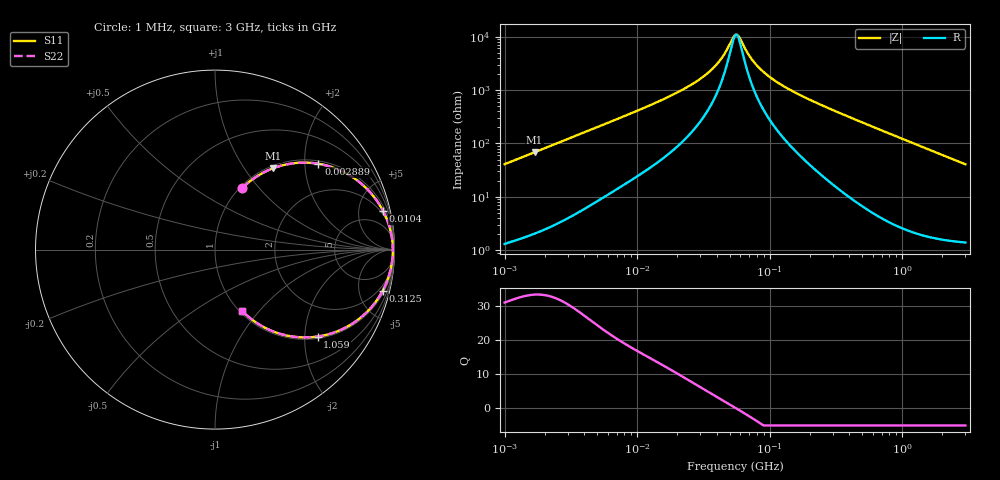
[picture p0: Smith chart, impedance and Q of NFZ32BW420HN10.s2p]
! NFZ32BW420HN10
# Hz S RI R 50
!Freq.(Hz) S11(Real) S11(Imag) S21(Real) S21(Imag) S12(Real) S12(Imag) S22(Real) S22(Imag)
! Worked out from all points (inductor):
!   401 points, 1 MHz to 3 GHz, reference 50 ohm
!   read as one part in series: L = 6.49 uH near 1.041 MHz
!   highest Q = 33.4 at 1.683 MHz (marker M1), where L = 6.48 uH
!   self-resonance near 55.88 MHz
!   S11 on the Smith chart (normalised r, x): 1 MHz: 1.03, +0.82; 2.889 MHz: 1.08, +2.34; 10.4 MHz: 1.52, +8.51; 312.5 MHz: 1.31, -8.08; 1.059 GHz: 1.05, -2.31; 3 GHz: 1.03, -0.82
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1000000  0.1517 0.3429  0.8483 -0.3429  0.8483 -0.3429  0.1517 0.3429
1682724  0.3243 0.4534  0.6757 -0.4534  0.6757 -0.4534  0.3243 0.4534
2888807  0.5761 0.4783  0.4239 -0.4783  0.4239 -0.4783  0.5761 0.4783
3823119  0.6992 0.441  0.3008 -0.441  0.3008 -0.441  0.6992 0.441
6180806  0.8513 0.3336  0.1487 -0.3336  0.1487 -0.3336  0.8513 0.3336
1.040059e7  0.9361 0.2161  0.0639 -0.2161  0.0639 -0.2161  0.9361 0.2161
1.461624e7  0.9634 0.1539  0.0366 -0.1539  0.0366 -0.1539  0.9634 0.1539
2.41077e7  0.9827 0.0839  0.0173 -0.0839  0.0173 -0.0839  0.9827 0.0839
3.456417e7  0.9885 0.0448  0.0115 -0.0448  0.0115 -0.0448  0.9885 0.0448
4.307715e7  0.9902 0.0238  0.00978 -0.0238  0.00978 -0.0238  0.9902 0.0238
5.477226e7  0.991 0.00198  0.00904 -0.00198  0.00904 -0.00198  0.991 0.00198
5.816196e7  0.991 -0.00341  0.00902 0.00341  0.00902 0.00341  0.991 -0.00341
7.248696e7  0.9905 -0.0234  0.00948 0.0234  0.00948 0.0234  0.9905 -0.0234
9.216659e7  0.9889 -0.0466  0.0111 0.0466  0.0111 0.0466  0.9889 -0.0466
1.295243e8  0.9839 -0.0839  0.0161 0.0839  0.0161 0.0839  0.9839 -0.0839
2.094008e8  0.9669 -0.1523  0.0331 0.1523  0.0331 0.1523  0.9669 -0.1523
3.124888e8  0.9344 -0.2288  0.0656 0.2288  0.0656 0.2288  0.9344 -0.2288
5.154121e8  0.8457 -0.3483  0.1543 0.3483  0.1543 0.3483  0.8457 -0.3483
8.005644e8  0.6982 -0.4483  0.3018 0.4483  0.3018 0.4483  0.6982 -0.4483
1.059487e9  0.5712 -0.4845  0.4288 0.4845  0.4288 0.4845  0.5712 -0.4845
1.645649e9  0.3596 -0.4683  0.6404 0.4683  0.6404 0.4683  0.3596 -0.4683
3e9  0.1511 -0.3414  0.8489 0.3414  0.8489 0.3414  0.1511 -0.3414
